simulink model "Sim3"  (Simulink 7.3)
settings: Solver=ode45  StartTime=0.0  StopTime=200  RelTol=1e-3
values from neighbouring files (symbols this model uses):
  Kp = om^2    (= 1.44)    [run.m]
  Kp3 = [0.3042  3.4539  0.5105  0.0711 -0.2670]    [run.m]
  Kr = 2*zt*om    (= 0.336)    [run.m]
undefined symbols (not defined in the file or in its folder): An, Bn, Cn, Dn

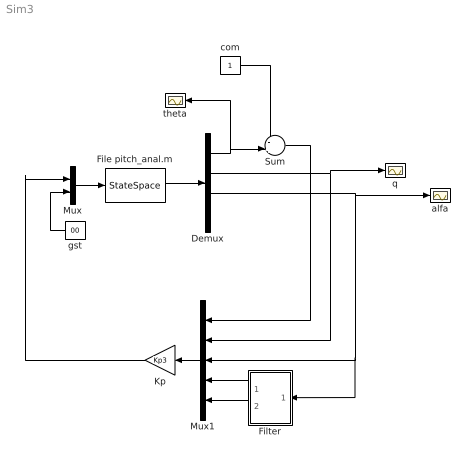
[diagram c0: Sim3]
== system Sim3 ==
  Demux : Demux
  File pitch_anal.m : StateSpace  A=An  B=Bn  C=Cn  D=Dn
  Filter : Subsystem
  Kp : Gain  Gain=Kp3  Multiplication=Matrix(K*u)  ParameterDataType=sfix(16)  ParameterScaling=2^0  OutDataType=sfix(16)  OutScaling=2^0
  Mux : Mux  Inputs=2
  Mux1 : Mux  Inputs=5
  Sum : Sum  Inputs=-+|  OutDataType=sfix(16)  OutScaling=2^0
  alfa : Scope
  com : Constant  OutDataType=sfix(16)  OutScaling=2^0
  gst : Constant  Value=00  OutDataType=sfix(16)  OutScaling=2^0
  q : Scope
  theta : Scope
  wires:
  Mux/1 -> File pitch_anal.m/1
  Demux/2 -> q/1, Mux1/2
  Sum/1 -> Mux1/1
  Demux/1 -> Sum/2, theta/1
  com/1 -> Sum/1
  gst/1 -> Mux/2
  Kp/1 -> Mux/1
  File pitch_anal.m/1 -> Demux/1
  Demux/3 -> alfa/1, Filter/1(a), Mux1/3
  Mux1/1 -> Kp/1
  Filter/1(x1) -> Mux1/4
  Filter/2(x2) -> Mux1/5

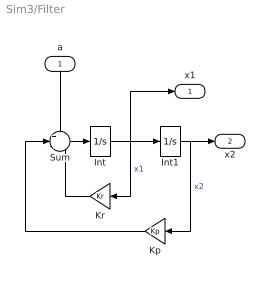
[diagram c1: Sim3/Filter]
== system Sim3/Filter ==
  a : Inport  OutDataType=sfix(16)  OutScaling=2^0
  Int : Integrator
  Int1 : Integrator
  Kp : Gain  Gain=Kp  ParameterDataType=sfix(16)  ParameterScaling=2^0  OutDataType=sfix(16)  OutScaling=2^0
  Kr : Gain  Gain=Kr  ParameterDataType=sfix(16)  ParameterScaling=2^0  OutDataType=sfix(16)  OutScaling=2^0
  Sum : Sum  Inputs=+--  OutDataType=sfix(16)  OutScaling=2^0
  x1 : Outport  OutDataType=sfix(16)  OutScaling=2^0
  x2 : Outport  Port=2  OutDataType=sfix(16)  OutScaling=2^0
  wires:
  Int/1 -> Int1/1, Kr/1, x1/1  "x1"
  Sum/1 -> Int/1
  Int1/1 -> Kp/1, x2/1  "x2"
  Kr/1 -> Sum/3
  Kp/1 -> Sum/2
  a/1 -> Sum/1
